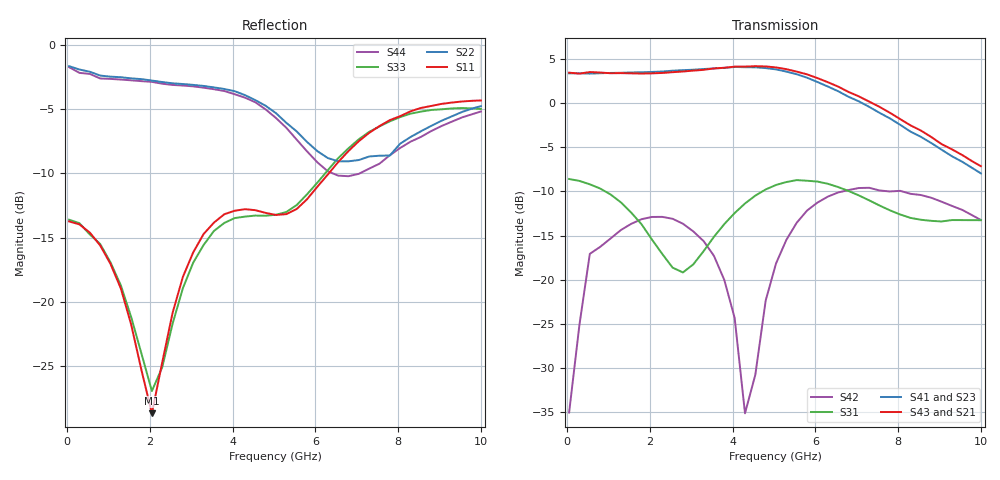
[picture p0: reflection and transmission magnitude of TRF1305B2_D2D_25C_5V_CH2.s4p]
!Created with skrf (http://scikit-rf.org).
! PORT[1] = INP
! PORT[2] = OUTM
! PORT[3] = INM
! PORT[4] = OUTP
# Hz S MA R 50.0
!freq magS11 angS11 magS12 angS12 magS13 angS13
! magS14 angS14
! magS21 angS21 magS22 angS22 magS23 angS23
! magS24 angS24
! magS31 angS31 magS32 angS32 magS33 angS33
! magS34 angS34
! magS41 angS41 magS42 angS42 magS43 angS43
! magS44 angS44
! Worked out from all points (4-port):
!   41 points, 50 MHz to 10 GHz, reference 50 ohm
!   strongest paths, dB at 50 MHz, 2.55 GHz, 5.05 GHz, 7.55 GHz, 10 GHz:
!     S43: 3.4, 3.5, 4.0, -0.4, -7.1
!     S41: 3.4, 3.7, 3.8, -1.1, -8.0
!     S21: 3.4, 3.5, 4.0, -0.8, -7.0
!     S23: 3.5, 3.5, 3.7, -1.4, -8.2
!     S31: -8.6, -18.6, -9.3, -11.6, -13.3
!     S42: -35.0, -13.1, -18.2, -9.9, -13.2
!   lowest |S11| = -28.7 dB at 2.05 GHz (marker M1), VSWR 1.08, Z = 53.7 + j0.77 ohm
!   |S11| at or under -10 dB: start of sweep to 6.322 GHz
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5e7  0.2057 -1.3  0.004265 48.8  0.3737 -2.3  0.003469 123.8
     1.479 177.5  0.828 177.6  1.493 -2.5  0.01425 102.4
     0.3717 -2.4  0.001542 96.9  0.2089 -2.2  0.002876 24.4
     1.474 -2.2  0.01771 110.6  1.487 177.5  0.8208 177.4
2.05e9  0.0368 11.2  0.04261 -23.3  0.1717 -101.0  0.03238 -44.6
        1.471 77.9  0.7278 109.4  1.483 -99.7  0.2308 2.7
        0.169 -103.7  0.02974 -48.9  0.04493 1.9  0.04591 -22.9
        1.501 -99.8  0.2266 3.8  1.474 77.6  0.7194 110.1
3.55e9  0.2036 32.9  0.05394 -73.0  0.172 111.7  0.03905 -122.9
        1.558 1.4  0.6845 67.8  1.556 -176.5  0.1362 -50.8
        0.1749 108.0  0.03556 -125.4  0.1889 35.7  0.05888 -74.8
        1.571 -176.7  0.1364 -47.8  1.571 1.5  0.6734 68.3
4.3e9  0.2296 15.2  0.06012 -96.8  0.2715 73.3  0.03737 -165.4
       1.604 -40.1  0.6386 47.7  1.576 142.0  0.01946 -108.1
       0.27 70.9  0.03383 -169.6  0.2148 20.9  0.06315 -97.8
       1.596 141.4  0.01752 -88.6  1.609 -39.8  0.6242 48.0
5.05e9  0.218 8.9  0.06804 -123.4  0.3529 43.2  0.03301 148.3
        1.58 -84.0  0.543 29.7  1.535 97.7  0.1289 84.0
        0.3439 41.8  0.03079 148.7  0.2184 16.9  0.07022 -123.9
        1.552 96.8  0.1236 79.3  1.592 -84.1  0.5199 29.4
6.55e9  0.35 6.8  0.07617 178.7  0.3487 -6.0  0.01796 57.9
        1.215 -171.5  0.3528 23.1  1.16 8.9  0.3216 26.2
        0.3347 -4.3  0.01733 61.6  0.3625 11.7  0.07897 -179.8
        1.167 8.5  0.3117 24.8  1.24 -170.9  0.3103 26.0
1e10  0.6088 -90.5  0.07769 54.4  0.2012 -37.6  0.01198 103.5
      0.4449 27.5  0.5785 4.3  0.3874 -157.5  0.2324 -50.7
      0.2172 -37.0  0.00683 99.7  0.5641 -80.2  0.07881 59.0
      0.4 -163.1  0.2177 -50.8  0.4392 29.8  0.5513 8.6
